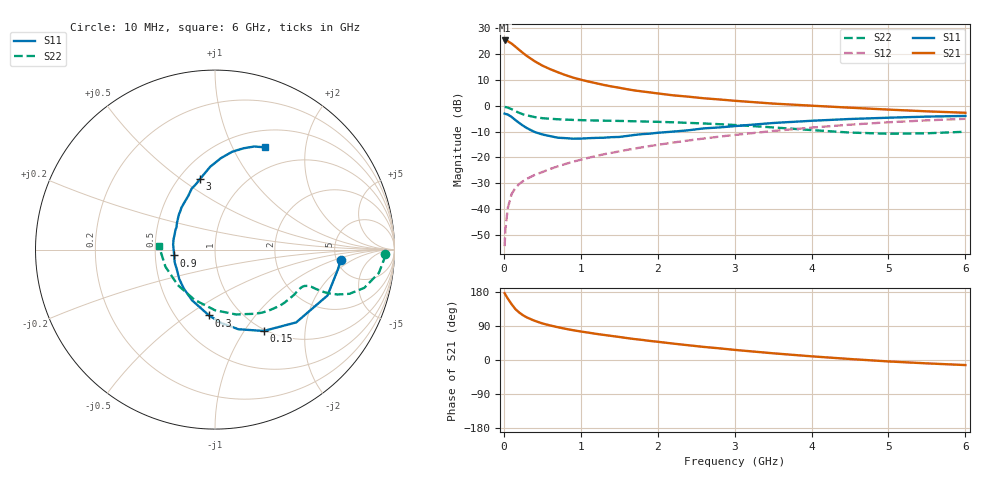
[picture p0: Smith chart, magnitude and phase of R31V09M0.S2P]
! SIEMENS Small Signal Semiconductors
! BFR181
! Si NPN RF Bipolar Junction Transistor in SOT23
! VCE = 1 V  IC = 9 mA
! Common Emitter S-Parameters:  May  1996
# GHz  S  MA  R  50
!  f  S11  S21  S12  S22
! GHz  MAG  ANG  MAG  ANG  MAG  ANG  MAG  ANG
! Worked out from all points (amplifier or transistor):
!   36 points, 10 MHz to 6 GHz, reference 50 ohm
!   highest |S21| = 25.3 dB at 10 MHz (marker M1)
!   |S21| within 3 dB of that: start of sweep to 173.8 MHz
!   unconditionally stable (mu >= 1): 456.7 MHz to 3.57 GHz
!   at 250 MHz: K = 0.72, MSG = 24.8 dB, |S12| = -29.2 dB
!   at 1.4 GHz: K = 1.22, MAG = 10.0 dB, |S12| = -18.3 dB
!   at 6 GHz: K = 0.98, MSG = 1.2 dB, |S12| = -5.1 dB
!   S11 on the Smith chart (normalised r, x): 10 MHz: 5.44, -1.24; 150 MHz: 0.98, -1.23; 300 MHz: 0.72, -0.61; 900 MHz: 0.63, -0.04; 3 GHz: 0.63, +0.59; 6 GHz: 0.71, +1.35
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0.01  0.703 -4.7  18.38 176.4  0.0019 85.7  0.9471 -1.6
0.02  0.6937 -9.1  18.21 172.7  0.0039 86.1  0.9435 -3.3
0.05  0.6769 -22.2  17.82 162.5  0.0102 79.4  0.9222 -8.1
0.1  0.6075 -41.9  16.02 147.5  0.0193 72.9  0.8582 -14.4
0.15  0.5283 -59.1  13.93 134.4  0.0255 65.4  0.7885 -18.2
0.2  0.4625 -73.6  12.07 125.2  0.0305 63.1  0.7275 -20.1
0.25  0.4105 -85.1  10.48 118.0  0.0346 61.3  0.6814 -21.0
0.3  0.3684 -95.2  9.192 112.2  0.0384 61.8  0.6505 -21.3
0.4  0.31 -114.4  7.291 103.5  0.0455 62.0  0.603 -21.3
0.5  0.2776 -128.9  5.987 96.5  0.0518 63.4  0.5742 -21.1
0.6  0.2579 -140.6  5.125 91.3  0.0594 64.4  0.5585 -21.2
0.7  0.2398 -152.3  4.463 86.6  0.0667 65.6  0.5469 -21.7
0.9  0.2295 -171.8  3.507 78.6  0.0822 66.5  0.5309 -22.8
1.1  0.235 173.0  2.94 72.2  0.098 67.4  0.5206 -24.7
1.3  0.2399 159.8  2.523 66.2  0.1146 67.5  0.5134 -27.0
1.6  0.2592 144.8  2.089 57.9  0.1392 66.8  0.5038 -31.0
2.2  0.3154 122.2  1.59 43.3  0.1932 63.8  0.4776 -40.9
3  0.4022 102.0  1.247 26.7  0.2713 57.3  0.4232 -57.6
3.5  0.4625 93.3  1.1 17.7  0.3238 52.1  0.38 -72.0
4.5  0.5531 80.1  0.916 2.6  0.4293 39.3  0.3019 -112.4
5.5  0.6149 69.1  0.778 -8.9  0.5203 25.0  0.2922 -160.8
6  0.6346 63.8  0.73 -13.4  0.5574 17.4  0.3132 176.3
